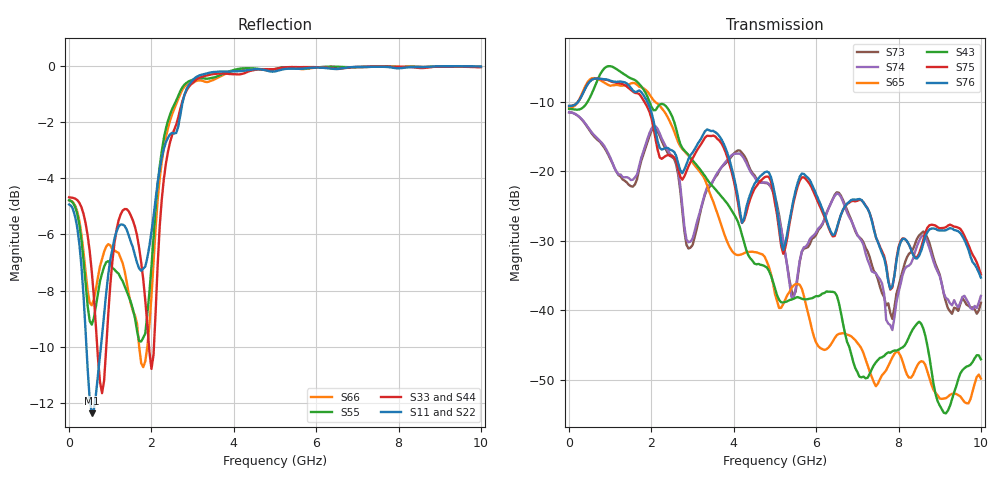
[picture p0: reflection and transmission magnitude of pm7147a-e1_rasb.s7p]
# GHz S DB R 50
! S-Parameters data
! Freq  dbS11  angS11  dbS12  angS12  dbS13  angS13  dbS14  angS14
!  dbS15  angS15  dbS16  angS16  dbS17  angS17  dbS21  angS21
!  dbS22  angS22  dbS23  angS23  dbS24  angS24  dbS25  angS25
!  dbS26  angS26  dbS27  angS27  dbS31  angS31  dbS32  angS32
!  dbS33  angS33  dbS34  angS34  dbS35  angS35  dbS36  angS36
!  dbS37  angS37  dbS41  angS41  dbS42  angS42  dbS43  angS43
!  dbS44  angS44  dbS45  angS45  dbS46  angS46  dbS47  angS47
!  dbS51  angS51  dbS52  angS52  dbS53  angS53  dbS54  angS54
!  dbS55  angS55  dbS56  angS56  dbS57  angS57  dbS61  angS61
!  dbS62  angS62  dbS63  angS63  dbS64  angS64  dbS65  angS65
!  dbS66  angS66  dbS67  angS67  dbS71  angS71  dbS72  angS72
!  dbS73  angS73  dbS74  angS74  dbS75  angS75  dbS76  angS76
!  dbS77  angS77
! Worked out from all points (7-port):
!   279 points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, 1 Hz to 10 GHz, reference 50 ohm
!   strongest paths, dB at 1 Hz, 7.943 MHz, 3.05 GHz, 6.55 GHz, 10 GHz:
!     S76: -10.6, -10.6, -16.8, -27.2, -35.3
!     S75: -10.6, -10.6, -17.6, -27.2, -34.8
!     S43: -11.0, -11.0, -18.8, -38.9, -47.1
!     S65: -10.9, -10.9, -19.2, -43.4, -49.8
!     S74: -11.5, -11.5, -28.6, -23.3, -37.9
!     S73: -11.5, -11.5, -29.5, -23.1, -38.9
!   lowest |S11| = -12.4 dB at 550 MHz (marker M1), VSWR 1.63, Z = 30.6 + j1.47 ohm
!   |S11| at or under -10 dB: 420.7 MHz to 771.5 MHz (350.8 MHz wide, 58.8 % of centre)
